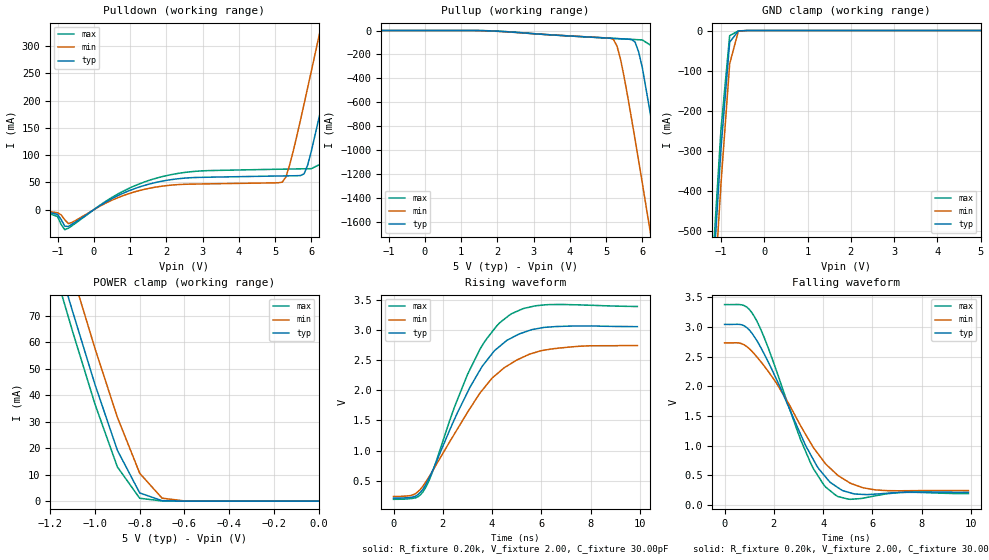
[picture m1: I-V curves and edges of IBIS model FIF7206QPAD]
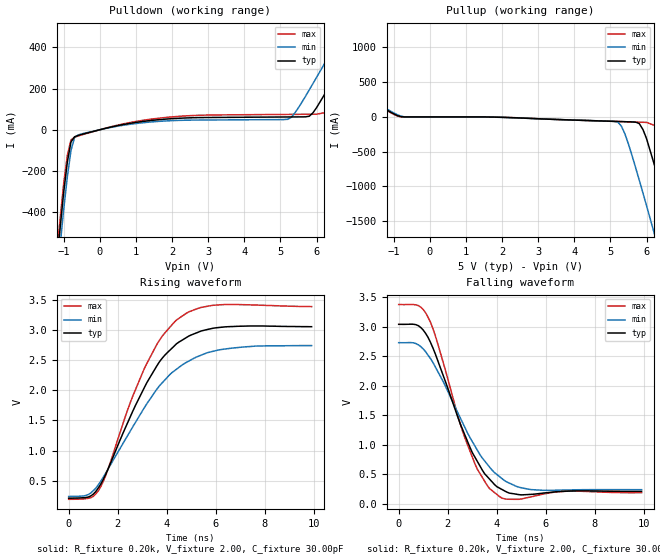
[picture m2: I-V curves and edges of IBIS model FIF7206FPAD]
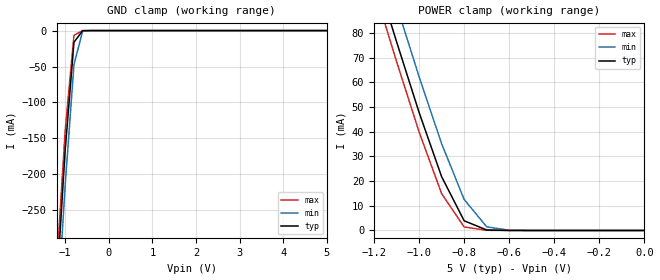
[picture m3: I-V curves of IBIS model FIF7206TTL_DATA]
| IBIS file idt7206.ibs created by s2ibis2 version 1.1
| North Carolina State University Electronics Research Laboratory  1995
[IBIS ver]   2.1
[File name]   idt7206.ibs
[File Rev]   1.0
[Date]   09/14/98
[Source]   Integrated Device Technology, Inc.
[Notes]   1. Temperatures: typ=25C, min=70C, max=0C 2. Cemos8_5v
   process. 3. Ramp rates based on 50 ohm load.
[Copyright]   Copyright 1997, Integrated Device Technology, Inc.
|   Component idt7206
[Component]   idt7206
[Manufacturer]   Integrated Device Technology
[Package]
| variable   typ   min   max
R_pkg   0.75   0.60   0.90
L_pkg   8.10nH   8.30nH   9.90nH
C_pkg   0.53pF   0.46pF   0.60pF
[Pin]  signal_name   model_name   R_pin   L_pin   C_pin
1   NC   NC
2   WINL   FIF7206TTL_RW
3   D8   FIF7206TTL_DATA
4   D3   FIF7206TTL_DATA
5   D2   FIF7206TTL_DATA
6   D1   FIF7206TTL_DATA
7   D0   FIF7206TTL_DATA
8   XIL   FIF7206TTL_XIL
9   FFL   FIF7206FPAD
10   Q0   FIF7206QPAD
11   Q1   FIF7206QPAD
12   NC   NC
13   Q2   FIF7206QPAD
14   Q3   FIF7206QPAD
15   Q8   FIF7206QPAD
16   GND   GND
17   NC   NC
18   RINL   FIF7206TTL_RW
19   Q4   FIF7206QPAD
20   Q5   FIF7206QPAD
21   Q6   FIF7206QPAD
22   Q7   FIF7206QPAD
23   XOLHFL   FIF7206FPAD
24   EFL   FIF7206FPAD
25   RSL   FIF7206TTL_RST
26   FLRTL   FIF7206TTL_FLRT
27   NC   NC
28   D7   FIF7206TTL_DATA
29   D6   FIF7206TTL_DATA
30   D5   FIF7206TTL_DATA
31   D4   FIF7206TTL_DATA
32   VCC   POWER
| Models and submodels in the file (7): FIF7206QPAD (3-state), FIF7206FPAD (Output), FIF7206TTL_DATA (Input), FIF7206TTL_FLRT (Input), FIF7206TTL_RST (Input), FIF7206TTL_RW (Input), FIF7206TTL_XIL (Input)
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| FIN  FIN   dummy_model
| QIN  QIN   dummy_model
| QOEL QOEL   dummy_model
|   Model FIF7206QPAD
[Model]   FIF7206QPAD
Model_type   3-state
Polarity   Non-Inverting
Enable   Active-Low
Vmeas =  1.500V
C_comp   3.00pF   NA   NA
[Temperature Range]   25.00   70.00   0.000
[Voltage Range]   5.00V   4.50V   5.50V
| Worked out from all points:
|   slope of the pulldown table from 0 to 0.75 V, typ, clamps not added: 26.4 ohm
|   GND clamp passes 1 mA (typ) near -0.58 V on its own axis
|   POWER clamp passes 1 mA (typ) near -0.73 V on its own axis
|   rising waveform, R_fixture 0.20k, V_fixture 2.00, C_fixture 30.00pF: 20-80 % time 2.06ns typ, 2.42ns min, 1.87ns max; typ from 0.212 V to 3.05 V
|   falling waveform, R_fixture 0.20k, V_fixture 2.00, C_fixture 30.00pF: 20-80 % time 1.89ns typ, 2.21ns min, 1.68ns max; typ from 3.04 V to 0.212 V
[Pulldown]
| voltage   I(typ)   I(min)   I(max)
-5V       0A         0A         -1mA
-1.4V     -2mA       -2mA       -2.6mA
-800mV    -30.31mA   -18.46mA   -36.64mA
1.7V      49.86mA    41.4mA     57.4mA
5.2V      62.01mA    50.65mA    74.43mA
5.4V      62.22mA    81.43mA    74.66mA
5.8V      65.73mA    194mA      75.11mA
6V        107mA      254mA      75.33mA
6.4V      223mA      376mA      88.69mA
6.8V      345mA      500mA      199mA
7.2V      469mA      625mA      320mA
10V       1.346A     1.502A     1.196A
[Pullup]
| voltage   I(typ)   I(min)   I(max)
-5V       0A         0A         0A
1.5V      -479uA     -1.046mA   -164uA
5.2V      -65.7mA    -73.43mA   -65.97mA
5.3V      -67.33mA   -129mA     -67.59mA
5.4V      -68.96mA   -242mA     -69.22mA
5.8V      -96.33mA   -913mA     -75.69mA
6V        -312mA     -1.278A    -78.93mA
6.4V      -1.007A    -2.022A    -157mA
6.8V      -1.749A    -2.775A    -777mA
7.2V      -2.503A    -3.533A    -1.515A
7.6V      -3.261A    -4.294A    -2.268A
10V       -7.849A    -8.884A    -6.848A
[GND_clamp]
| voltage   I(typ)   I(min)   I(max)
-5V       -7.848A    -7.925A    -7.806A
-1.2V     -639mA     -728mA     -591mA
-1V       -293mA     -380mA     -245mA
-800mV    -29.04mA   -82.96mA   -12.82mA
-600mV    -1.086mA   -1.823mA   -995uA
-400mV    -11.58nA   -1.65uA    -4.45nA
5V        50nA       1.299uA    50nA
[POWER_clamp]
| voltage   I(typ)   I(min)   I(max)
-5V       1.28A      1.292A     1.274A
-1.2V     100mA      114mA      92.9mA
-1.1V     71.67mA    85.58mA    64.09mA
-1V       44.09mA    57.71mA    36.65mA
-900mV    19.26mA    31.72mA    12.95mA
-800mV    3.093mA    10.54mA    1.086mA
-700mV    173uA      1.126mA    65.17uA
-600mV    6.6uA      79.66uA    270nA
0V        50nA       45nA       55nA
[Ramp]
| variable   typ   min   max
dV/dt_r   1.00/1.13n   0.85/1.43n   1.15/0.97n
dV/dt_f   1.68/1.85n   1.37/2.24n   1.96/1.61n
R_load = 50.00
[Rising Waveform]
R_fixture = 0.20k
V_fixture = 2.00
C_fixture = 30.00pF
R_dut = 0.75
L_dut = 8.10nH
C_dut = 0.53pF
| time   V(typ)   V(min)   V(max)
0s        212mV      240mV      193mV
900ps     246mV      290mV      218mV
1.3ns     430mV      475mV      385mV
1.6ns     681mV      673mV      667mV
3ns       1.964V     1.632V     2.258V
3.7ns     2.449V     2.05V      2.805V
4.4ns     2.759V     2.341V     3.147V
5.2ns     2.947V     2.538V     3.342V
6ns       3.033V     2.657V     3.409V
9.9ns     3.054V     2.741V     3.388V
[Falling Waveform]
R_fixture = 0.20k
V_fixture = 2.00
C_fixture = 30.00pF
R_dut = 0.75
L_dut = 8.10nH
C_dut = 0.53pF
| time   V(typ)   V(min)   V(max)
0s        3.045V     2.733V     3.38V
800ps     3.021V     2.7V       3.362V
1.2ns     2.843V     2.551V     3.184V
2.1ns     2.125V     2.059V     2.271V
3.5ns     843mV      1.041V     701mV
4.1ns     472mV      693mV      302mV
4.5ns     320mV      536mV      167mV
5.3ns     183mV      336mV      99.94mV
6.1ns     181mV      254mV      151mV
9.9ns     212mV      241mV      190mV
|   Model FIF7206FPAD
[Model]   FIF7206FPAD
Model_type   Output
Vmeas =  1.500V
C_comp   3.00pF   NA   NA
[Temperature Range]   25.00   70.00   0.000
[Voltage Range]   5.00V   4.50V   5.50V
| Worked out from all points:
|   slope of the pulldown table from 0 to 0.75 V, typ, clamps not added: 26.4 ohm
|   rising waveform, R_fixture 0.20k, V_fixture 2.00, C_fixture 30.00pF: 20-80 % time 2.03ns typ, 2.41ns min, 1.86ns max; typ from 0.212 V to 3.05 V
|   falling waveform, R_fixture 0.20k, V_fixture 2.00, C_fixture 30.00pF: 20-80 % time 1.58ns typ, 1.88ns min, 1.4ns max; typ from 3.04 V to 0.211 V
[Pulldown]
| voltage   I(typ)   I(min)   I(max)
-5V       -7.848A    -7.925A    -7.807A
-1.4V     -1.005A    -1.092A    -957mA
-1V       -301mA     -385mA     -258mA
-800mV    -59.36mA   -101mA     -49.46mA
-600mV    -27.75mA   -25.16mA   -30.34mA
5.2V      62.01mA    50.65mA    74.43mA
5.8V      65.73mA    194mA      75.11mA
6.4V      223mA      376mA      88.69mA
6.8V      345mA      500mA      199mA
7.2V      469mA      625mA      320mA
8V        719mA      875mA      568mA
10V       1.346A     1.502A     1.196A
[Pullup]
| voltage   I(typ)   I(min)   I(max)
-5V       1.28A      1.292A     1.274A
-1.4V     160mA      174mA      152mA
-800mV    3.093mA    10.54mA    1.086mA
5.2V      -65.7mA    -73.43mA   -65.97mA
5.4V      -68.96mA   -242mA     -69.22mA
5.8V      -96.33mA   -913mA     -75.69mA
6V        -312mA     -1.278A    -78.93mA
6.4V      -1.007A    -2.022A    -157mA
6.8V      -1.749A    -2.775A    -777mA
7.2V      -2.503A    -3.533A    -1.515A
7.6V      -3.261A    -4.294A    -2.268A
10V       -7.849A    -8.884A    -6.848A
[Ramp]
| variable   typ   min   max
dV/dt_r   1.00/1.14n   0.85/1.34n   1.15/0.95n
dV/dt_f   1.68/1.18n   1.37/1.41n   1.97/1.04n
R_load = 50.00
[Rising Waveform]
R_fixture = 0.20k
V_fixture = 2.00
C_fixture = 30.00pF
R_dut = 0.75
L_dut = 8.10nH
C_dut = 0.53pF
| time   V(typ)   V(min)   V(max)
0s        212mV      240mV      193mV
800ps     231mV      272mV      209mV
1.2ns     377mV      429mV      328mV
1.5ns     599mV      622mV      578mV
2.4ns     1.46V      1.248V     1.673V
3.1ns     2.059V     1.723V     2.376V
3.7ns     2.473V     2.074V     2.83V
4.4ns     2.773V     2.351V     3.167V
6.2ns     3.044V     2.675V     3.418V
9.9ns     3.054V     2.741V     3.387V
[Falling Waveform]
R_fixture = 0.20k
V_fixture = 2.00
C_fixture = 30.00pF
R_dut = 0.75
L_dut = 8.10nH
C_dut = 0.53pF
| time   V(typ)   V(min)   V(max)
0s        3.045V     2.733V     3.38V
800ps     3.022V     2.697V     3.362V
1.2ns     2.821V     2.52V      3.162V
1.6ns     2.421V     2.24V      2.706V
2.6ns     1.266V     1.38V      1.238V
3.1ns     797mV      986mV      687mV
3.7ns     421mV      626mV      260mV
4.1ns     269mV      465mV      126mV
5.4ns     161mV      241mV      118mV
9.9ns     211mV      240mV      190mV
|   Model FIF7206TTL_DATA
[Model]   FIF7206TTL_DATA
Model_type   Input
Vinl =  0.000V
Vinh =  3.000V
Vmeas =  1.500V
C_comp   3.00pF   NA   NA
[Temperature Range]   25.00   70.00   0.000
[Voltage Range]   5.00V   4.50V   5.50V
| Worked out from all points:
|   GND clamp passes 1 mA (typ) near -0.61 V on its own axis
|   POWER clamp passes 1 mA (typ) near -0.72 V on its own axis
[GND_clamp]
| voltage   I(typ)   I(min)   I(max)
-5V       -4.399A    -4.442A    -4.375A
-1.2V     -360mA     -410mA     -332mA
-1V       -165mA     -214mA     -138mA
-800mV    -16.2mA    -47.25mA   -6.498mA
-600mV    -99.37uA   -546uA     -20.34uA
5V        50nA       1.822uA    50nA
[POWER_clamp]
| voltage   I(typ)   I(min)   I(max)
-5V       1.327A     1.34A      1.32A
-1.2V     106mA      121mA      98.35mA
-1.1V     76.53mA    91.28mA    68.48mA
-1V       47.85mA    62.33mA    39.94mA
-900mV    21.81mA    35.18mA    14.95mA
-800mV    3.94mA     12.59mA    1.419mA
-700mV    207uA      1.478mA    70.87uA
-600mV    6.867uA    94.52uA    358nA
0V        50nA       45nA       55nA
